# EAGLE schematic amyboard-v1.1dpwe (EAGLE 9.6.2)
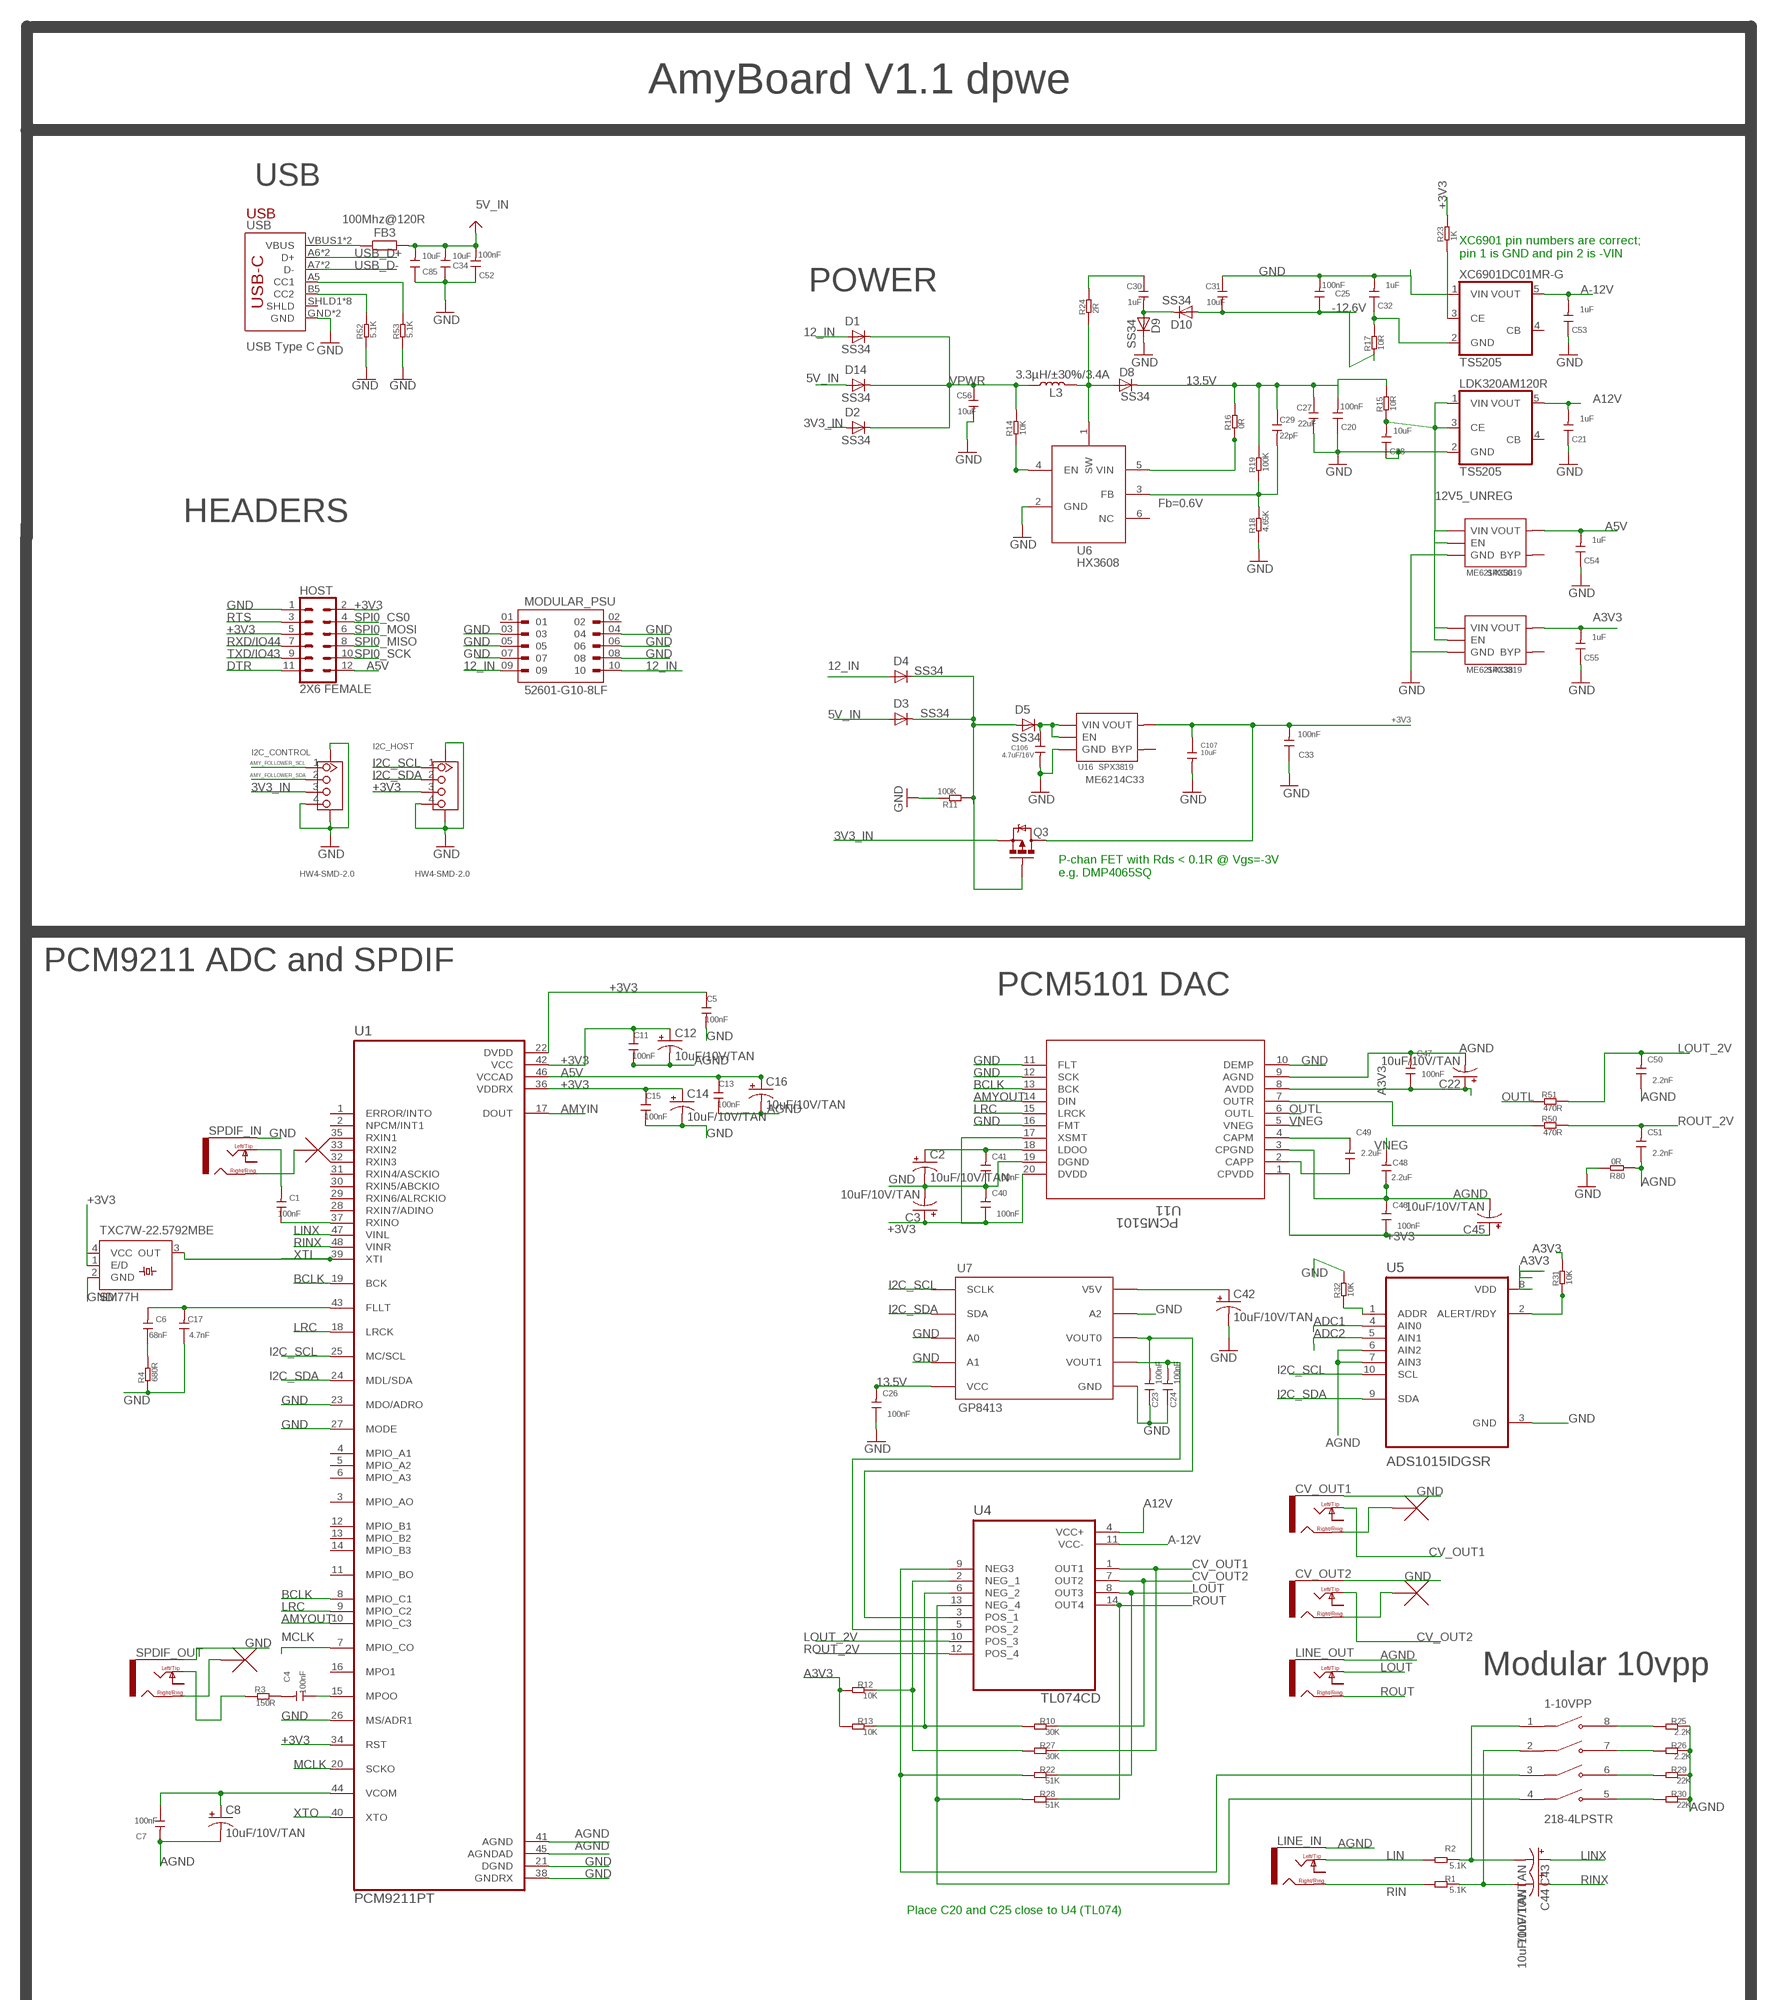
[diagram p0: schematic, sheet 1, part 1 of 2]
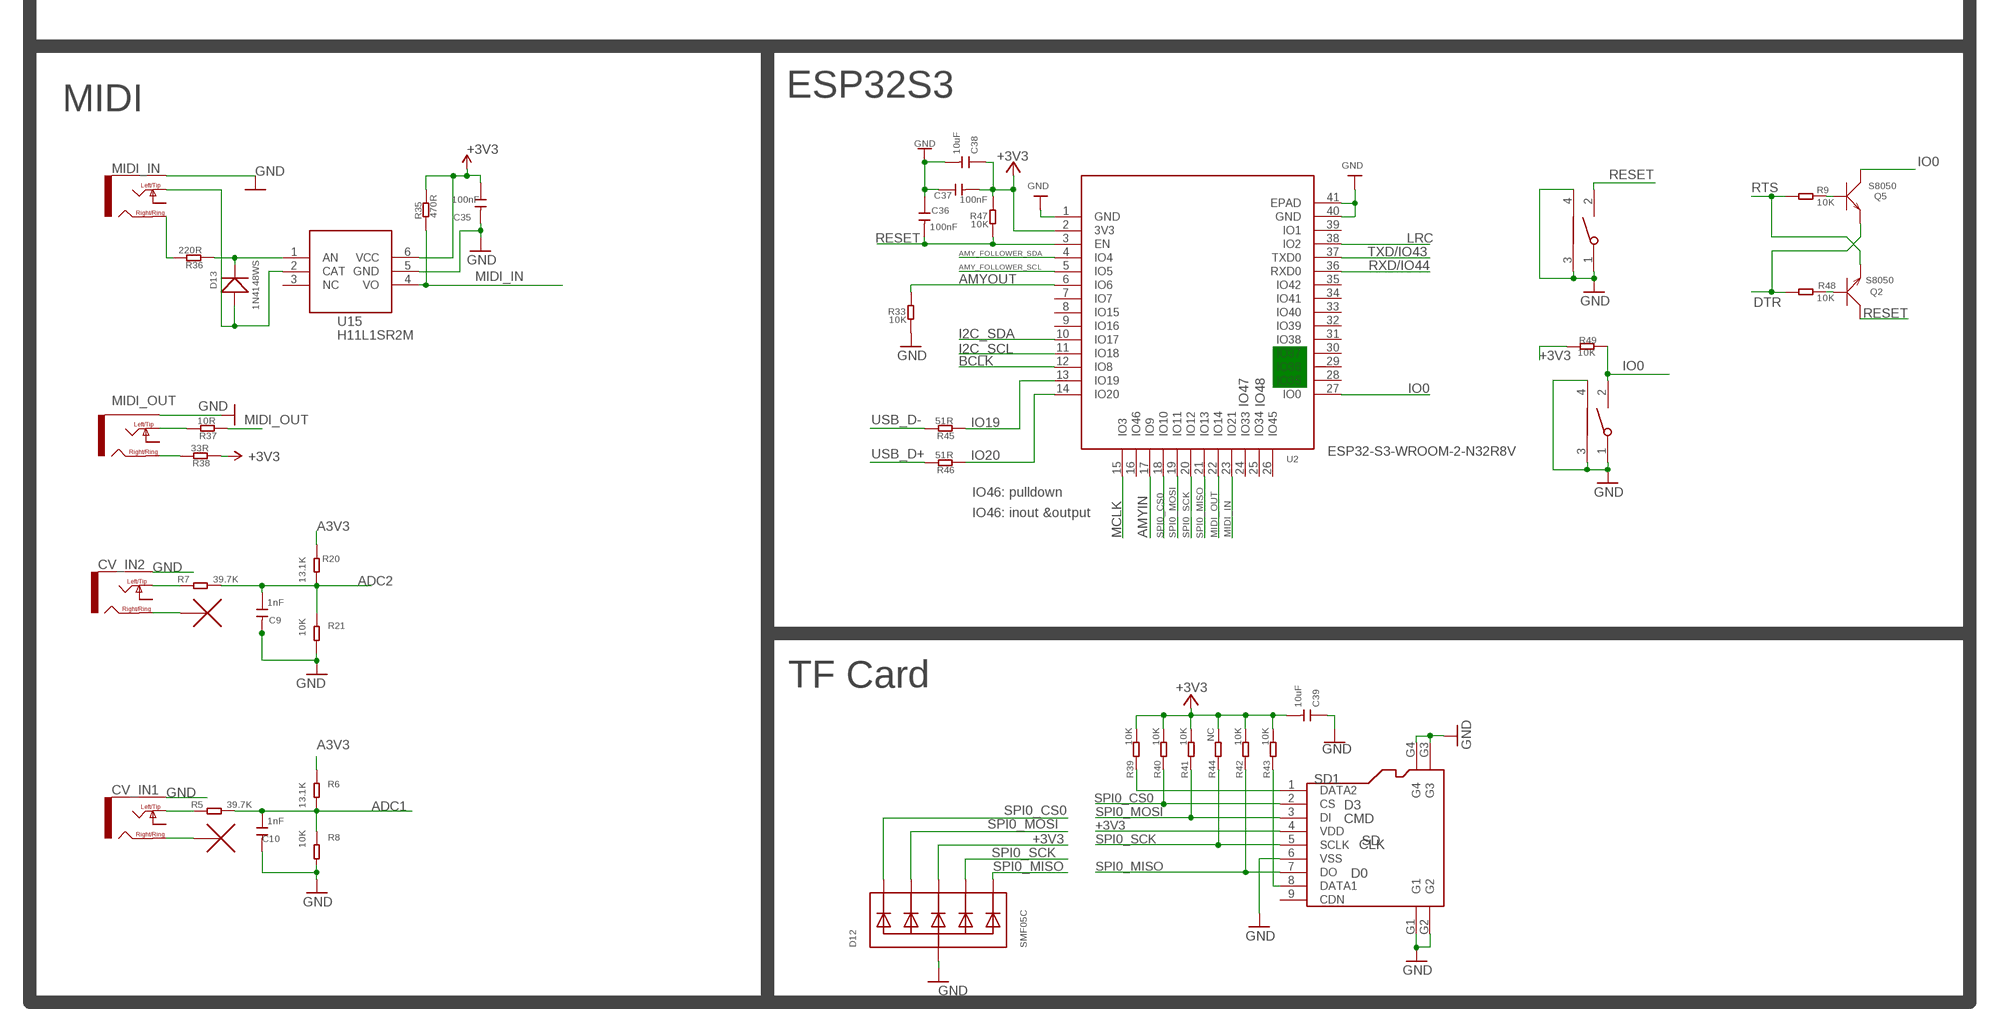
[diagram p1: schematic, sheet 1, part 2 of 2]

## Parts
1-10VPP  218-4LPSTR  [SW_218-4LPSTR]
BOOT  TS24CA  [2*4*3.5MM]
C1  100nF  DISCRETE_C-0402  [DISCRETE_C0402]
C2  10uF/10V/TAN  CPOL-USSMCZ  [SMC_Z]
C3  10uF/10V/TAN  CPOL-USSMCZ  [SMC_Z]
C4  100nF  DISCRETE_C-0402  [DISCRETE_C0402]
C5  100nF  DISCRETE_C-0402  [DISCRETE_C0402]
C6  68nF  DISCRETE_C-0402  [DISCRETE_C0402]
C7  100nF  DISCRETE_C-0402  [DISCRETE_C0402]
C8  10uF/10V/TAN  CPOL-USSMCZ  [SMC_Z]
C9  1nF  DISCRETE_C-0402  [DISCRETE_C0402]
C10  1nF  DISCRETE_C-0402  [DISCRETE_C0402]
C11  100nF  DISCRETE_C-0402  [DISCRETE_C0402]
C12  10uF/10V/TAN  CPOL-USSMCZ  [SMC_Z]
C13  100nF  DISCRETE_C-0402  [DISCRETE_C0402]
C14  10uF/10V/TAN  CPOL-USSMCZ  [SMC_Z]
C15  100nF  DISCRETE_C-0402  [DISCRETE_C0402]
C16  10uF/10V/TAN  CPOL-USSMCZ  [SMC_Z]
C17  4.7nF  DISCRETE_C-0402  [DISCRETE_C0402]
C20  100nF  DISCRETE_C-0402  [DISCRETE_C0402]
C21  1uF  DISCRETE_C-0402  [DISCRETE_C0402]
C22  10uF/10V/TAN  CPOL-USSMCZ  [SMC_Z]
C23  100nF  DISCRETE_C-0402  [DISCRETE_C0402]
C24  100nF  DISCRETE_C-0402  [DISCRETE_C0402]
C25  100nF  DISCRETE_C-0402  [DISCRETE_C0402]
C26  100nF  DISCRETE_C-0402  [DISCRETE_C0402]
C27  22uF  CAP-0603  [C0603]
C28  10uF  DISCRETE_C-0402  [DISCRETE_C0402]
C29  22pF  CAP-0603  [C0603]
C30  1uF  CAP-0603  [C0603]
C31  10uF  CAP-0603  [C0603]
C32  1uF  DISCRETE_C-0402  [DISCRETE_C0402]
C33  100nF  DISCRETE_C-0402  [DISCRETE_C0402]
C34  10uF  DISCRETE_C-0603  [DISCRETE_C0603]
C35  100nF  DISCRETE_C-0402  [DISCRETE_C0402]
C36  100nF  DISCRETE_C-0402  [DISCRETE_C0402]
C37  100nF  DISCRETE_C-0402  [DISCRETE_C0402]
C38  10uF  DISCRETE_C-0603  [DISCRETE_C0603]
C39  10uF  DISCRETE_C-0603  [DISCRETE_C0603]
C40  100nF  DISCRETE_C-0402  [DISCRETE_C0402]
C41  100nF  DISCRETE_C-0402  [DISCRETE_C0402]
C42  10uF/10V/TAN  CPOL-USSMCZ  [SMC_Z]
C43  10uF/10V/TAN  CPOL-USSMCZ  [SMC_Z]
C44  10uF/10V/TAN  CPOL-USSMCZ  [SMC_Z]
C45  10uF/10V/TAN  CPOL-USSMCZ  [SMC_Z]
C46  100nF  DISCRETE_C-0402  [DISCRETE_C0402]
C47  100nF  DISCRETE_C-0402  [DISCRETE_C0402]
C48  2.2uF  DISCRETE_C-0402  [DISCRETE_C0402]
C49  2.2uF  DISCRETE_C-0402  [DISCRETE_C0402]
C50  2.2nF  DISCRETE_C-0402  [DISCRETE_C0402]
C51  2.2nF  DISCRETE_C-0402  [DISCRETE_C0402]
C52  100nF  DISCRETE_C-0402  [DISCRETE_C0402]
C53  1uF  DISCRETE_C-0402  [DISCRETE_C0402]
C54  1uF  DISCRETE_C-0402  [DISCRETE_C0402]
C55  1uF  DISCRETE_C-0402  [DISCRETE_C0402]
C56  10uF  CAP-0603  [C0603]
C85  10uF  DISCRETE_C-0603  [DISCRETE_C0603]
C106  4.7uF/16V  C-0603  [0603]
C107  10uF  C-0603  [0603]
CV_IN1  NV-PJ3410_STEREO  [NV-PJ3410_SOCKET]
CV_IN2  NV-PJ3410_STEREO  [NV-PJ3410_SOCKET]
CV_OUT1  NV-PJ3410_STEREO  [NV-PJ3410_SOCKET]
CV_OUT2  NV-PJ3410_STEREO  [NV-PJ3410_SOCKET]
D1  SS34  DIODE-DO-214AC  [DO-214AC]
D2  SS34  DIODE-DO-214AC  [DO-214AC]
D3  SS34  DIODE-DO-214AC  [DO-214AC]
D4  SS34  DIODE-DO-214AC  [DO-214AC]
D5  SS34  DIODE-DO-214AC  [DO-214AC]
D8  SS34  DIODE-DO-214AC  [DO-214AC]
D9  SS34  DIODE-DO-214AC  [DO-214AC]
D10  SS34  DIODE-DO-214AC  [DO-214AC]
D12  SMF05C  TVSARRAY_5LANE  [SOT363]
D13  1N4148WS  D'0805'  [SOD323]
D14  SS34  DIODE-DO-214AC  [DO-214AC]
FB3  100Mhz@120R  R-EU_R0805  [R0805]
HOST  2X6 FEMALE  CONN_06X2PTH_FEMALE  [2X6]
I2C_CONTROL  HW4-SMD-2.0  GROVE-CONNECTOR-SMD'90D'  [HW4-SMD-2.0-90D]
I2C_HOST  HW4-SMD-2.0  GROVE-CONNECTOR-SMD'90D'  [HW4-SMD-2.0-90D]
L3  3.3µH/±30%/3.4A  INDUCTOR-CR54-3.3UH  [CR54]
LDK320AM120R  TS5205  [SOT25]
LINE_IN  NV-PJ3410_STEREO  [NV-PJ3410_SOCKET]
LINE_OUT  NV-PJ3410_STEREO  [NV-PJ3410_SOCKET]
ME6214C33  SPX3819  [SOT23-5]
ME6214C50  SPX3819  [SOT23-5]
MIDI_IN  NV-PJ3410_STEREO  [NV-PJ3410_SOCKET]
MIDI_OUT  NV-PJ3410_STEREO  [NV-PJ3410_SOCKET]
MODULAR_PSU  52601-G10-8LF  [AMPHENOL_52601-G10-8LF]
PCM5101  U11  PCM5101APW  [PW20_TEX]
Q2  S8050  TRANSISTOR-NPN-SOT23  [SOT23]
Q3  AO3407  MOSFET-PCHANNEL  [SOT23-3]
Q5  S8050  TRANSISTOR-NPN-SOT23  [SOT23]
R1  5.1K  DISCRETE_R-0402  [DISCRETE_R0402]
R2  5.1K  DISCRETE_R-0402  [DISCRETE_R0402]
R3  150R  DISCRETE_R-0402  [DISCRETE_R0402]
R4  680R  DISCRETE_R-0402  [DISCRETE_R0402]
R5  39.7K  DISCRETE_R-0402  [DISCRETE_R0402]
R6  13.1K  DISCRETE_R-0402  [DISCRETE_R0402]
R7  39.7K  DISCRETE_R-0402  [DISCRETE_R0402]
R8  10K  DISCRETE_R-0402  [DISCRETE_R0402]
R9  10K  DISCRETE_R-0402  [DISCRETE_R0402]
R10  30K  DISCRETE_R-0402  [DISCRETE_R0402]
R11  100K  DISCRETE_R-0402  [DISCRETE_R0402]
R12  10K  DISCRETE_R-0402  [DISCRETE_R0402]
R13  10K  DISCRETE_R-0402  [DISCRETE_R0402]
R14  10K  DISCRETE_R-0402  [DISCRETE_R0402]
R15  10R  DISCRETE_R-0402  [DISCRETE_R0402]
R16  0R  DISCRETE_R-0402  [DISCRETE_R0402]
R17  10R  DISCRETE_R-0402  [DISCRETE_R0402]
R18  4.65K  DISCRETE_R-0402  [DISCRETE_R0402]
R19  100K  DISCRETE_R-0402  [DISCRETE_R0402]
R20  13.1K  DISCRETE_R-0402  [DISCRETE_R0402]
R21  10K  DISCRETE_R-0402  [DISCRETE_R0402]
R22  51K  DISCRETE_R-0402  [DISCRETE_R0402]
R23  1K  DISCRETE_R-0402  [DISCRETE_R0402]
R24  2R  DISCRETE_R-0402  [DISCRETE_R0402]
R25  2.2K  DISCRETE_R-0402  [DISCRETE_R0402]
R26  2.2K  DISCRETE_R-0402  [DISCRETE_R0402]
R27  30K  DISCRETE_R-0402  [DISCRETE_R0402]
R28  51K  DISCRETE_R-0402  [DISCRETE_R0402]
R29  22K  DISCRETE_R-0402  [DISCRETE_R0402]
R30  22K  DISCRETE_R-0402  [DISCRETE_R0402]
R31  10K  DISCRETE_R-0402  [DISCRETE_R0402]
R32  10K  DISCRETE_R-0402  [DISCRETE_R0402]
R33  10K  DISCRETE_R-0402  [DISCRETE_R0402]
R35  470R  DISCRETE_R-0402  [DISCRETE_R0402]
R36  220R  DISCRETE_R-0402  [DISCRETE_R0402]
R37  10R  DISCRETE_R-0402  [DISCRETE_R0402]
R38  33R  DISCRETE_R-0402  [DISCRETE_R0402]
R39  10K  DISCRETE_R-0402  [DISCRETE_R0402]
R40  10K  DISCRETE_R-0402  [DISCRETE_R0402]
R41  10K  DISCRETE_R-0402  [DISCRETE_R0402]
R42  10K  DISCRETE_R-0402  [DISCRETE_R0402]
R43  10K  DISCRETE_R-0402  [DISCRETE_R0402]
R44  NC  DISCRETE_R-0402  [DISCRETE_R0402]
R45  51R  DISCRETE_R-0402  [DISCRETE_R0402]
R46  51R  DISCRETE_R-0402  [DISCRETE_R0402]
R47  10K  DISCRETE_R-0402  [DISCRETE_R0402]
R48  10K  DISCRETE_R-0402  [DISCRETE_R0402]
R49  10K  DISCRETE_R-0402  [DISCRETE_R0402]
R50  470R  DISCRETE_R-0402  [DISCRETE_R0402]
R51  470R  DISCRETE_R-0402  [DISCRETE_R0402]
R52  5.1K  DISCRETE_R-0402  [DISCRETE_R0402]
R53  5.1K  DISCRETE_R-0402  [DISCRETE_R0402]
R80  0R  DISCRETE_R-0603  [DISCRETE_R0603]
RST  TS24CA  [2*4*3.5MM]
SD1  SD  HOLDER-MICROSD-9P  [9P-SMD-W/-RING]
SPDIF_IN  NV-PJ3410_STEREO  [NV-PJ3410_SOCKET]
SPDIF_OUT  NV-PJ3410_STEREO  [NV-PJ3410_SOCKET]
TXC7W-22.5792MBE  SM77H  [SM77H]
U1  PCM9211PT  [QFP50P900X900X160-48N]
U2  ESP32­S2­SOLO  [ESP32-­S2-­SOLO]
U4  TL074CD  [SOIC127P600X175-14N]
U5  ADS1015IDGSR  [SOP50P490X110-10N]
U6  HX3608  [SOT-23-6]
U7  GP8413  [SOIC-10]
U15  H11L1SR2M  [SOP-6-2.54MM]
U16  SPX3819  [SOT23-5]
U$1  NC_MARKER  (no package)
U$2  NC_MARKER  (no package)
U$3  NC_MARKER  (no package)
U$4  NC_MARKER  (no package)
U$5  NC_MARKER  (no package)
U$6  NC_MARKER  (no package)
USB  USB-C  USB_C5  [USB-C-16P-5]
XC6901DC01MR-G  TS5205  [SOT25]

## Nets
3V3_IN: D2.A I2C_CONTROL.3 Q3.2(S)
5V_IN: C34.2 C52.2 C85.2 D3.A D14.A FB3.2 ; supply symbol labelled VBUS
12_IN: D1.A D4.A MODULAR_PSU.09 MODULAR_PSU.10
12V5_UNREG: C28.2 LDK320AM120R.1(VIN) LDK320AM120R.3(CE) ME6214C33.1(VIN) ME6214C33.3(EN) ME6214C50.1(VIN) ME6214C50.3(EN) R15.2
13.5V: C20.2 C26.2 C27.1 C29.1 D8.C R15.1 R16.1 R19.1 U7.5(VCC)
+3V3: C3.+ C5.1 C11.1 C12.+ C14.+ C15.1 C33.2 C35.1 C37.2 C38.1 C39.2 C40.1 C45.+ C46.1 C107.1 D12.4(C3) HOST.2 HOST.5 I2C_HOST.3 PCM5101.1(CPVDD) PCM5101.17(XSMT) PCM5101.20(DVDD) Q3.3(D) R23.1 R35.1 R38.2 R39.2 R40.2 R41.2 R42.2 R43.2 R44.2 R47.2 R49.2 SD1.4(VDD) TXC7W-22.5792MBE.1(E/D) TXC7W-22.5792MBE.4(VCC) U1.22(DVDD) U1.34(RST) U1.36(VDDRX) U1.42(VCC) U2.2(3V3) U15.6(VCC) U16.5(VOUT)
-12.6V: C25.1 R17.2
A3V3: C22.+ C47.1 C55.2 ME6214C33.5(VOUT) PCM5101.8(AVDD) R6.2 R12.2 R13.2 R20.2 R31.1 U5.8(VDD)
A5V: C13.1 C16.+ C54.2 HOST.12 ME6214C50.5(VOUT) U1.46(VCCAD)
A12V: C21.2 LDK320AM120R.5(VOUT) U4.4(VCC+)
A-12V: C53.2 U4.11(VCC-) XC6901DC01MR-G.5(VOUT)
ADC1: C10.1 R5.1 R6.1 R8.2 U5.4(AIN0)
ADC2: C9.1 R7.1 R20.1 R21.2 U5.5(AIN1)
AGND: C7.2 C8.- C11.2 C12.- C13.2 C16.- C22.- C45.- C46.2 C47.2 C48.1 C50.1 C51.1 LINE_IN.GND(EARTH) LINE_OUT.GND(EARTH) PCM5101.3(CPGND) PCM5101.9(AGND) R25.1 R26.1 R29.1 R30.1 R80.1 U1.41(AGND) U1.45(AGNDAD) U5.6(AIN2) U5.7(AIN3)
AMY_FOLLOWER_SCL: I2C_CONTROL.1 U2.5(IO5)
AMY_FOLLOWER_SDA: I2C_CONTROL.2 U2.4(IO4)
AMYIN: U1.17(DOUT) U2.17(IO9)
AMYOUT: PCM5101.14(DIN) R33.2 U1.10(MPIO_C3) U2.6(IO6)
BCLK: PCM5101.13(BCK) U1.8(MPIO_C1) U1.19(BCK) U2.12(IO8)
CV_OUT1: CV_OUT1.LEFT/TIP(TIP) R27.1 U4.1(OUT1)
CV_OUT2: CV_OUT2.LEFT/TIP(TIP) R10.1 U4.7(OUT2)
DTR: HOST.11 Q5.2(E) R48.2
ENABLE: R14.2 U6.4(EN)
GND: BOOT.1 BOOT.3 BOOT.4 C2.- C3.- C5.2 C9.2 C10.2 C14.- C15.2 C17.1 C20.1 C21.1 C23.1 C24.1 C25.2 C26.1 C27.2 C28.1 C31.1 C32.2 C33.1 C34.1 C35.2 C36.1 C37.1 C38.2 C39.1 C40.2 C41.1 C42.- C52.1 C53.1 C54.1 C55.1 C56.2 C85.1 C106.2 C107.2 CV_IN1.GND(EARTH) CV_IN2.GND(EARTH) CV_OUT1.GND(EARTH) CV_OUT2.GND(EARTH) D9.C D12.2(A) HOST.1 I2C_CONTROL.4 I2C_CONTROL.SS1 I2C_CONTROL.SS2 I2C_HOST.4 I2C_HOST.SS1 I2C_HOST.SS2 LDK320AM120R.2(GND) ME6214C33.2(GND) ME6214C50.2(GND) MIDI_IN.GND(EARTH) MIDI_OUT.GND(EARTH) MODULAR_PSU.03 MODULAR_PSU.04 MODULAR_PSU.05 MODULAR_PSU.06 MODULAR_PSU.07 MODULAR_PSU.08 PCM5101.10(DEMP) PCM5101.11(FLT) PCM5101.12(SCK) PCM5101.16(FMT) PCM5101.19(DGND) R4.2 R8.1 R11.1 R18.2 R21.1 R32.1 R33.1 R52.2 R53.2 R80.2 RST.1 RST.3 RST.4 SD1.6(VSS) SD1.G1 SD1.G2 SD1.G3 SD1.G4 SPDIF_IN.GND(EARTH) SPDIF_OUT.GND(EARTH) TXC7W-22.5792MBE.2(GND) U1.21(DGND) U1.23(MDO/ADRO) U1.26(MS/ADR1) U1.27(MODE) U1.38(GNDRX) U2.1(GND) U2.40(GND) U2.41(EPAD) U5.3(GND) U6.2(GND) U7.3(A0) U7.4(A1) U7.6(GND) U7.9(A2) U15.5(GND) U16.2(GND) USB.GND USB.GND2(GND) XC6901DC01MR-G.1(VIN)
I2C_SCL: I2C_HOST.1 U1.25(MC/SCL) U2.11(IO18) U5.10(SCL) U7.1(SCLK)
I2C_SDA: I2C_HOST.2 U1.24(MDL/SDA) U2.10(IO17) U5.9(SDA) U7.2(SDA)
IO0: BOOT.2 Q5.3(C) R49.1 U2.27(IO0)
IO19: R45.2 U2.13(IO19)
IO20: R46.2 U2.14(IO20)
LIN: LINE_IN.LEFT/TIP(TIP) R2.2
LINX: C43.+ U1.47(VINL)
LOUT: LINE_OUT.LEFT/TIP(TIP) R22.1 U4.8(OUT3)
LOUT_2V: C50.2 R51.1 U4.10(POS_3)
LRC: PCM5101.15(LRCK) U1.9(MPIO_C2) U1.18(LRCK) U2.38(IO2)
MCLK: U1.7(MPIO_CO) U1.20(SCKO) U2.15(IO3)
MIDI_IN: R35.2 U2.23(IO21) U15.4(VO)
MIDI_OUT: R37.2 U2.22(IO14)
N$1: C1.1 U1.37(RXINO)
N$2: C4.2 R3.1
N$3: C4.1 U1.15(MPOO)
N$4: 1-10VPP.1 C43.- R2.1
N$5: 1-10VPP.2 C44.- R1.1
N$6: C7.1 C8.+ U1.44(VCOM)
N$7: C6.2 C17.2 U1.43(FLLT)
N$8: C6.1 R4.1
N$9: SPDIF_OUT.RIGHT/RING(RING) U$1.P$1
N$10: SPDIF_IN.RIGHT/RING(RING) U$2.P$1
N$11: CV_OUT1.RIGHT/RING(RING) U$3.P$1
N$12: CV_OUT2.RIGHT/RING(RING) U$4.P$1
N$13: CV_IN2.LEFT/TIP(TIP) R7.2
N$14: CV_IN2.RIGHT/RING(RING) U$6.P$1
N$15: C32.1 R17.1 XC6901DC01MR-G.2(GND)
N$16: C31.2 D10.A
N$17: CV_IN1.RIGHT/RING(RING) U$5.P$1
N$18: C23.2 U4.3(POS_1) U7.8(VOUT0)
N$19: CV_IN1.LEFT/TIP(TIP) R5.2
N$20: C24.2 U4.5(POS_2) U7.7(VOUT1)
N$21: D8.A L3.P$2 R24.2 U6.1(SW)
N$22: C42.+ U7.10(V5V)
N$23: D3.C D4.C D5.A Q3.1(G) R11.2
N$24: C106.1 D5.C U16.1(VIN) U16.3(EN)
N$26: C29.2 R18.1 R19.2 U6.3(FB)
N$27: C30.1 R24.1
N$28: R16.2 U6.5(VIN)
N$29: C30.2 D9.A D10.C
N$30: R23.2 XC6901DC01MR-G.3(CE)
N$31: R10.2 R13.1 U4.6(NEG_2)
N$33: R12.1 R27.2 U4.2(NEG_1)
N$34: Q2.1(B) R48.1
N$35: 1-10VPP.5 R30.2
N$36: 1-10VPP.6 R29.2
N$37: Q5.1(B) R9.1
N$38: R53.1 USB.A5(CC1)
N$39: R52.1 USB.B5(CC2)
N$40: 1-10VPP.8 R25.2
N$41: 1-10VPP.7 R26.2
N$42: FB3.1 USB.VBUS1(VBUS) USB.VBUS2(VBUS)
N$43: R31.2 U5.2(ALERT/RDY)
N$44: 1-10VPP.3 R22.2 U4.9(NEG3)
N$45: 1-10VPP.4 R28.2 U4.13(NEG_4)
N$46: R32.2 U5.1(ADDR)
N$48: C2.+ C41.2 PCM5101.18(LDOO)
N$50: PCM5101.7(OUTR) R50.2
N$51: C49.2 PCM5101.4(CAPM)
N$52: C49.1 PCM5101.2(CAPP)
N$55: D13.+ MIDI_IN.LEFT/TIP(TIP) U15.2(CAT)
N$56: MIDI_IN.RIGHT/RING(RING) R36.1
N$57: D13.- R36.2 U15.1(AN)
N$58: MIDI_OUT.LEFT/TIP(TIP) R37.1
N$59: MIDI_OUT.RIGHT/RING(RING) R38.1
N$75: R39.1 SD1.1(DATA2)
N$77: R43.1 SD1.8(DATA1)
OUTL: PCM5101.6(OUTL) R51.2
RESET: C36.2 Q2.3(C) R47.1 RST.2 U2.3(EN)
RIN: LINE_IN.RIGHT/RING(RING) R1.2
RINX: C44.+ U1.48(VINR)
ROUT: LINE_OUT.RIGHT/RING(RING) R28.1 U4.14(OUT4)
ROUT_2V: C51.2 R50.1 U4.12(POS_4)
RTS: HOST.3 Q2.2(E) R9.2
RXD/IO44: HOST.7 U2.36(RXD0)
SPDIFIN_SIGNAL: C1.2 SPDIF_IN.LEFT/TIP(TIP)
SPDIFOUT_SIGNAL: R3.2 SPDIF_OUT.LEFT/TIP(TIP)
SPI0_CS0: D12.1(C1) HOST.4 R40.1 SD1.2(CS) U2.18(IO10)
SPI0_MISO: D12.6(C5) HOST.8 R42.1 SD1.7(DO) U2.21(IO13)
SPI0_MOSI: D12.3(C2) HOST.6 R41.1 SD1.3(DI) U2.19(IO11)
SPI0_SCK: D12.5(C4) HOST.10 R44.1 SD1.5(SCLK) U2.20(IO12)
TXD/IO43: HOST.9 U2.37(TXD0)
USB_D+: R46.1 USB.A6(D+) USB.B6(D+)
USB_D-: R45.1 USB.A7(D-) USB.B7(D-)
VNEG: C48.2 PCM5101.5(VNEG)
VPWR: C56.1 D1.C D2.C D14.C L3.P$1 R14.1
XTI: TXC7W-22.5792MBE.3(OUT) U1.39(XTI)
XTO: U1.40(XTO)
Unconnected: CV_IN1.SWITCH(TIP-NORM) CV_IN2.SWITCH(TIP-NORM) CV_OUT1.SWITCH(TIP-NORM) CV_OUT2.SWITCH(TIP-NORM) LDK320AM120R.4(CB) LINE_IN.SWITCH(TIP-NORM) LINE_OUT.SWITCH(TIP-NORM) ME6214C33.4(BYP) ME6214C50.4(BYP) MIDI_IN.SWITCH(TIP-NORM) MIDI_OUT.SWITCH(TIP-NORM) MODULAR_PSU.01 MODULAR_PSU.02 SD1.9(CDN) SPDIF_IN.SWITCH(TIP-NORM) SPDIF_OUT.SWITCH(TIP-NORM) U1.1(ERROR/INTO) U1.2(NPCM/INT1) U1.3(MPIO_AO) U1.4(MPIO_A1) U1.5(MPIO_A2) U1.6(MPIO_A3) U1.11(MPIO_BO) U1.12(MPIO_B1) U1.13(MPIO_B2) U1.14(MPIO_B3) U1.16(MPO1) U1.28(RXIN7/ADINO) U1.29(RXIN6/ALRCKIO) U1.30(RXIN5/ABCKIO) U1.31(RXIN4/ASCKIO) U1.32(RXIN3) U1.33(RXIN2) U1.35(RXIN1) U2.7(IO7) U2.8(IO15) U2.9(IO16) U2.16(IO46) U2.24(IO33) U2.25(IO34) U2.26(IO45) U2.28(IO35) U2.29(IO36) U2.30(IO37) U2.31(IO38) U2.32(IO39) U2.33(IO40) U2.34(IO41) U2.35(IO42) U2.39(IO1) U6.6(NC) U15.3(NC) U16.4(BYP) USB.SHLD1(SHLD) USB.SHLD2(SHLD) USB.SHLD3(SHLD) USB.SHLD4(SHLD) USB.SHLD5(SHLD) USB.SHLD6(SHLD) USB.SHLD7(SHLD) USB.SHLD8(SHLD) XC6901DC01MR-G.4(CB)

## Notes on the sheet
- AmyBoard V1.1 dpwe
- USB
- USB
- XC6901 pin numbers are correct; 
  pin 1 is GND and pin 2 is -VIN
- POWER
- USB Type C
- Fb=0.6V
- HEADERS
- ME6214C33
- P-chan FET with Rds < 0.1R @ Vgs=-3V
  e.g. DMP4065SQ
- PCM9211 ADC and SPDIF
- PCM5101 DAC
- Modular 10vpp
- Place C20 and C25 close to U4 (TL074)
- ESP32S3
- MIDI
- IO47 | IO48
- ESP32-S3-WROOM-2-N32R8V
- IO46: pulldown
- IO46: inout &output
- TF Card
- D3
- CMD
- CLK
- D0

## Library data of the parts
1-10VPP = 218-4LPSTR:218-4LPSTR: Check availability; AVAILABILITY: In Stock; CHECK_PRICES: https://www.snapeda.com/parts/218-4LPSTR/CTS+Components/view-part/?ref=eda; DESCRIPTION: Dip Switch SPST 4 Position Surface Mount Slide (Standard) Actuator 25mA 24VDC; MF: CTS Electrocomponents; MP: 218-4LPSTR; PACKAGE: None; PRICE: None; SNAPEDA_LINK: https://www.snapeda.com/parts/218-4LPSTR/CTS+Components/view-part/?ref=snap
BOOT RST = sale:TS24CA
C1 C4-C7 C9-C11 C13 C15 C17 C20 C21 C23-C26 C28 C32-C41 C46-C55 C85 = A9G:DISCRETE_C*: Ceramic Capacitors
C2 C3 C8 C12 C14 C16 C22 C42-C45 = rcl:CPOL-US: POLARIZED CAPACITOR, American symbol
C27 C29-C31 C56 = Discrete-new:CAP: Ceramic Capacitors
C106 C107 = Discrete:C*: Ceramic Capacitors
CV_IN1 CV_IN2 CV_OUT1 CV_OUT2 LINE_IN LINE_OUT MIDI_IN MIDI_OUT SPDIF_IN SPDIF_OUT = PJ3410_sockets:NV-PJ3410_STEREO: PJ3410 socket stereo with switch
D1-D5 D8-D10 D14 = diode:DIODE-: DIODE
D12 = microbuilder:TVSARRAY_5LANE: Voltage Transient Suppressor Array SOT363 SMF05C - 100W 5V: Digikey - SMF05CT1GOSCT-ND
D13 = Discrete:D*
FB3 = rcl:R-EU_: RESISTOR, European symbol
HOST = SparkFun-Connectors:CONN_06X2: Multi connection point. Often used as Generic Header-pin footprint for 0.1 inch spaced/style header connections On any of the 0.1 inch spaced packages, you can populate with these: Break Away Headers - Straight (PRT-00116) Break Away Male Headers - Right Angle (PRT-00553) Female Headers (PRT-00115)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; PROD_ID: CONN-12423
I2C_CONTROL I2C_HOST = Connector-new:GROVE-CONNECTOR-SMD: 4P-SMD-2.0:320110030;4P-SMD-2.0-90D:320110032
L3 = SparkFun-Coils:INDUCTOR: Inductors; PROD_ID: NDUC-11157
LDK320AM120R XC6901DC01MR-G = v-reg:TS5205: 150mA Low Noise LDO Voltage Regulator with Enable TSC [Taiwan Semiconductor Company, Ltd] Source: http://www.taiwansemi.com .. 5205_0409c.pdf
ME6214C33 ME6214C50 U16 = IC:SPX3819
MODULAR_PSU = 52601-G10-8LF:52601-G10-8LF: Check availability; AVAILABILITY: In Stock; CHECK_PRICES: https://www.snapeda.com/parts/52601-G10-8LF/Amphenol+FCI/view-part/?ref=eda; DESCRIPTION: Conn; Rect; Header; SMT; Shroud; 2.54 mm; 2-Row; 10 Pos; Gold (30) Plate;Quickie | Amphenol FCI (Amphenol CS) 52601-G10-8LF; MF: Amphenol ICC; MP: 52601-G10-8LF; PACKAGE: None; PRICE: None; SNAPEDA_LINK: https://www.snapeda.com/parts/52601-G10-8LF/Amphenol+FCI/view-part/?ref=snap
PCM5101 = pcm5101apw:PCM5101APW; COPYRIGHT: Copyright (C) 2022 Ultra Librarian. All rights reserved.; DIGI-KEY_PART_NUMBER_1: PCM5101APW-ND; MANUFACTURER_PART_NUMBER: PCM5101APW; MFR_NAME: Texas Instruments
Q2 Q5 = Discrete:TRANSISTOR-NPN*: NPN audion
Q3 = User-Submitted:MOSFET-PCHANNEL: Generic PMOSFET IRLML2244 - TRANS-11153 (SOT-23 -20V -4.3A) (1.Gate 2.Source 3.Drain) FQP27P06 - COM-10349 (TO-220 -60V -27A) (1.Gate 2.Source 3.Drain); PROD_ID: TRANS-08285
R1-R33 R35-R53 R80 = A9G:DISCRETE_R*
SD1 = Connector:HOLDER-MICROSD-9P
TXC7W-22.5792MBE = crystal:SM77H: 3.3V CMOS Clock Oscillator Source: www.pletronics.com .. sm77h%203.3v.pdf; OC_FARNELL: unknown; OC_NEWARK: unknown
U1 = PCM9211PT:PCM9211PT: Check availability; AVAILABILITY: In Stock; CHECK_PRICES: https://www.snapeda.com/parts/PCM9211PT/Texas+Instruments/view-part/?ref=eda; DESCRIPTION: 216kHz Digital Audio Interface Transceiver (DIX) with Stereo ADC and Routing; MF: Texas Instruments; MP: PCM9211PT; PACKAGE: LQFP-48 Texas Instruments; PRICE: None; SNAPEDA_LINK: https://www.snapeda.com/parts/PCM9211PT/Texas+Instruments/view-part/?ref=snap
U2 = self:ESP32­S2­SOLO
U4 = TL074CD:TL074CD: Check availability; AVAILABILITY: In Stock; CHECK_PRICES: https://www.snapeda.com/parts/TL074CD/Texas+Instruments/view-part/?ref=eda; DESCRIPTION: Quad, 30-V, 3-MHz, high slew rate (13-V/µs), In to V+, JFET-input op amp; MF: Texas Instruments; MP: TL074CD; PACKAGE: SOIC-14 Texas Instruments; PRICE: None; SNAPEDA_LINK: https://www.snapeda.com/parts/TL074CD/Texas+Instruments/view-part/?ref=snap
U5 = ADS1015IDGSR:ADS1015IDGSR: Check availability; AVAILABILITY: In Stock; CHECK_PRICES: https://www.snapeda.com/parts/ADS1015IDGSR/Texas+Instruments/view-part/?ref=eda; DESCRIPTION: 12-bit, 3.3-kSPS, 4-channel, delta-sigma ADC with PGA, oscillator, VREF, comparator and I2C; MF: Texas Instruments; MP: ADS1015IDGSR; PACKAGE: VSSOP-10 Texas Instruments; PRICE: None; SNAPEDA_LINK: https://www.snapeda.com/parts/ADS1015IDGSR/Texas+Instruments/view-part/?ref=snap
U6 = self:HX3608
U7 = FL5160MX:GP8413: https://www.mouser.com/ProductDetail/ON-Semiconductor-Fairchild/FL5160MX?qs=%2fha2pyFaduhZ4yOtT1cFvr2BtPh63RpxkXQRTY8DgC4%3d Check availability; AVAILABILITY: In Stock; CHECK_PRICES: https://www.snapeda.com/parts/FL5160MX/Onsemi/view-part/?ref=eda; DESCRIPTION: Optocoupler Drive 1-CH 5.5V 10-Pin SOIC N T/R; MF: onsemi; MP: FL5160MX; PACKAGE: None; PRICE: None; SNAPEDA_LINK: https://www.snapeda.com/parts/FL5160MX/Onsemi/view-part/?ref=snap
U15 = sale:H11L1SR2M
U$1-U$6 = NC_MARKER:NC_MARKER
USB = USBC:USB_C: USB Type C 16Pin Connector Super Speed pins not available on the 16-pin purely SMD connector so this part is best for USB 2.0 implementations. D1 and D2 are tied together enabling D+/- no matter which way the cable is plugged into the connector. The two channel configuration pins (CC1/2) are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

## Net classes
0 default: width 0.152 mm, drill 0.305 mm, clearance 0.152 mm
